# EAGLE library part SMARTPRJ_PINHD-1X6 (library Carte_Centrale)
PIN HEADER
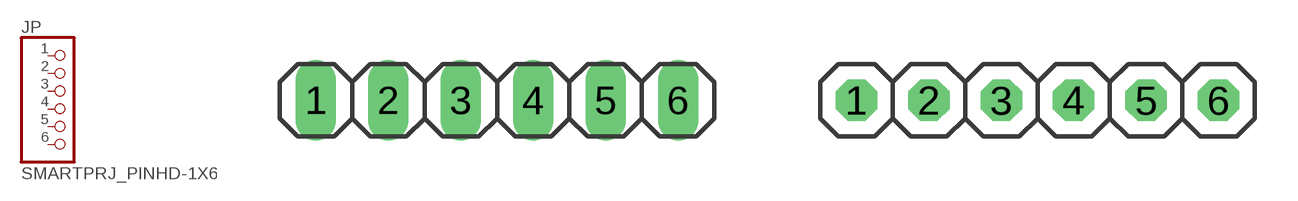
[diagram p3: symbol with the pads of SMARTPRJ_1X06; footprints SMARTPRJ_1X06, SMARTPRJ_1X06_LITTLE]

Designator prefix JP

## SMARTPRJ_PINHD-1X6  [SMARTPRJ_1X06]
1  1  pas
2  2  pas
3  3  pas
4  4  pas
5  5  pas
6  6  pas

## SMARTPRJ_PINHD-1X6LITTLE  [SMARTPRJ_1X06_LITTLE]
Pads as for SMARTPRJ_1X06

## SMARTPRJ_PINHD-1X6TH  [SMARTPRJ_1X06-TH]
Pads as for SMARTPRJ_1X06

## Footprint SMARTPRJ_1X06 (pad centres in mm)
PIN HEADER
drill 0.85 pad 1.422 long: 1 -6.35,0; 2 -3.81,0; 3 -1.27,0; 4 1.27,0; 5 3.81,0; 6 6.35,0

## Footprint SMARTPRJ_1X06_LITTLE (pad centres in mm)
drill 0.95 pad 1.422 octagon: 1 -6.35,0; 2 -3.81,0; 3 -1.27,0; 4 1.27,0; 5 3.81,0; 6 6.35,0

## Footprint SMARTPRJ_1X06-TH (pad centres in mm)
drill 0.95 pad 1.422 long: 1 -6.35,0; 2 -3.81,0; 3 -1.27,0; 4 1.27,0; 5 3.81,0; 6 6.35,0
